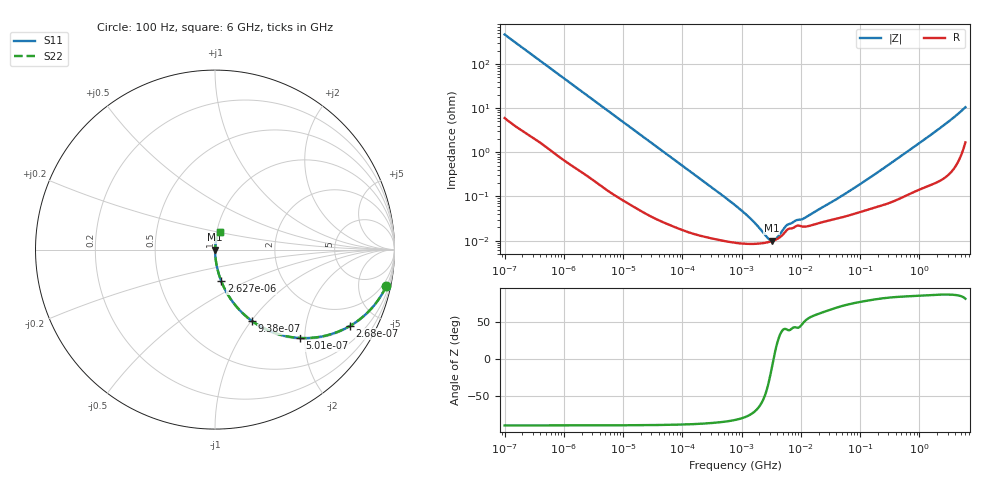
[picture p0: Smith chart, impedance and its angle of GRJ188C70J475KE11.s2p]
!Murata Part Number: GRJ188C70J475KE11
!These Parameters are Measured in Series Mode Connection
!Data Generated on Jun 19, 2026
!  o--ll--o
!Port1  Port2
!  o------o
!Operation Temp=25[degC], DC Bias Voltage=0[V]
!Freq. Start=100[Hz] Stop=6[GHz] 401[Steps]
# Hz S RI R 50
!Freq.(Hz) S11(Real) S11(Imag) S21(Real) S21(Imag) S12(Real) S12(Imag) S22(Real) S22(Imag)
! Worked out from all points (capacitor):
!   401 points, 100 Hz to 6 GHz, reference 50 ohm
!   read as one part in series: C = 3.4 uF near 109 Hz
!   lowest |Z| = 9.92 mohm at 3.246 MHz (marker M1)
!   series resonance near 3.469 MHz, so ESL is about 620 pH
!   S11 on the Smith chart (normalised r, x): 100 Hz: 1.12, -9.33; 268 Hz: 1.05, -3.51; 501 Hz: 1.03, -1.89; 938 Hz: 1.01, -1.01; 2.627 kHz: 1.01, -0.37; 6 GHz: 1.03, +0.21
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100  0.9537 -0.2039  0.0463 0.2039  0.0463 0.2039  0.9537 -0.2039
164  0.888 -0.3091  0.112 0.3091  0.112 0.3091  0.888 -0.3091
268  0.7519 -0.4252  0.2481 0.4252  0.2481 0.4252  0.7519 -0.4252
501  0.4712 -0.4922  0.5289 0.4922  0.5289 0.4922  0.4712 -0.4922
938  0.2075 -0.3986  0.7925 0.3986  0.7925 0.3986  0.2075 -0.3986
2008  0.0567 -0.2239  0.9433 0.2239  0.9433 0.2239  0.0567 -0.2239
2627  0.0347 -0.1757  0.9653 0.1757  0.9653 0.1757  0.0347 -0.1757
8047  0.00457 -0.0599  0.9954 0.0599  0.9954 0.0599  0.00457 -0.0599
40335  0.000436 -0.0122  0.9996 0.0122  0.9996 0.0122  0.000436 -0.0122
774597  8.96e-05 -0.00063  0.9999 0.00063  0.9999 0.00063  8.96e-05 -0.00063
1516199  8.42e-05 -0.000276  0.9999 0.000276  0.9999 0.000276  8.42e-05 -0.000276
2837864  9.24e-05 -6.05e-05  0.9999 6.05e-05  0.9999 6.05e-05  9.24e-05 -6.05e-05
3245845  9.72e-05 -1.99e-05  0.9999 1.99e-05  0.9999 1.99e-05  9.72e-05 -1.99e-05
3882480  0.000107 3.4e-05  0.9999 -3.4e-05  0.9999 -3.4e-05  0.000107 3.4e-05
5311619  0.00015 0.000128  0.9998 -0.000128  0.9998 -0.000128  0.00015 0.000128
6075234  0.000182 0.000146  0.9998 -0.000146  0.9998 -0.000146  0.000182 0.000146
1.087309e7  0.000208 0.000231  0.9998 -0.000231  0.9998 -0.000231  0.000208 0.000231
1.555665e7  0.000225 0.000349  0.9998 -0.000349  0.9998 -0.000349  0.000225 0.000349
5.960426e7  0.000361 0.00116  0.9996 -0.00116  0.9996 -0.00116  0.000361 0.00116
3.124326e8  0.00074 0.00531  0.9993 -0.00531  0.9993 -0.00531  0.00074 0.00531
1.95892e9  0.00301 0.0307  0.997 -0.0307  0.997 -0.0307  0.00301 0.0307
6e9  0.0266 0.0993  0.9734 -0.0993  0.9734 -0.0993  0.0266 0.0993
